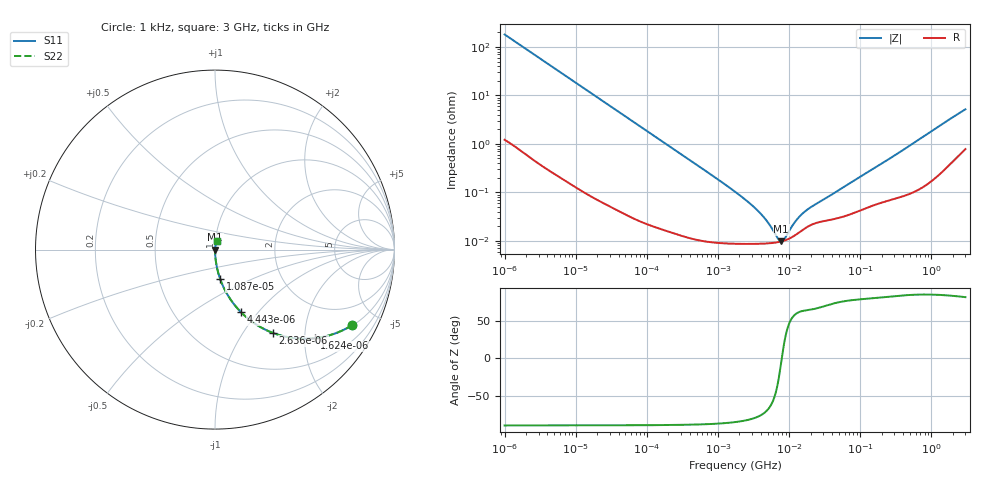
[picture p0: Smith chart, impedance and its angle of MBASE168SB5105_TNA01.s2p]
! MBASE168SB5105_TNA01  S-PARAMETER MODEL  ( Standard Model )
! Model Generated by TAIYO YUDEN Corporation (http://www.ty-top.com)
! Version 2.0
! TAIYO YUDEN Control No. 240510
! Copyright(c) 2012 TAIYO YUDEN CO.,LTD. All Rights Reserved.
! Product Description (link to TY-COMPAS)
! https://ds.yuden.co.jp/TYCOMPAS/or/detail?pn=MBASE168SB5105KTNA01&u=M
! Products Name : Multilayer Ceramic Capacitors
! Characteristics :
!  Capacitance : 1 [uF] , Rated Voltage : 16 [V] , TCC : X5R
!  Case Size : 1.6 x 0.8 / 0.063 x 0.031 [mm/inch] , Thickness : 0.8 / 0.031 [mm/inch]
!  (Conditions: Temperature = 25 [degC] , DC Bias Voltage = 0 [V])
! External Node Assignments :
!  1  o---| |---o  2
! GND o---------o GND
! Frequency Range : 1kHz  -  3GHz  [ 401 STEP ]
# MHZ S RI R 50
! Freq[MHz].  S11 Real  S11 Imag  S21 Real  S21 Imag  S12 Real  S12 Imag  S22 Real  S22 Imag
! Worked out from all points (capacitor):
!   401 points, 1 kHz to 3 GHz, reference 50 ohm
!   read as one part in series: C = 878 nF near 1.077 kHz
!   lowest |Z| = 9.73 mohm at 7.696 MHz (marker M1)
!   series resonance near 7.883 MHz, so ESL is about 460 pH
!   S11 on the Smith chart (normalised r, x): 1 kHz: 1.02, -3.62; 1.624 kHz: 1.02, -2.24; 2.636 kHz: 1.01, -1.38; 4.443 kHz: 1.01, -0.82; 10.87 kHz: 1.00, -0.34; 3 GHz: 1.02, +0.10
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0.001  0.7647 -0.4209  0.2353 0.4209  0.2353 0.4209  0.7647 -0.4209
0.001624  0.555 -0.4936  0.445 0.4936  0.445 0.4936  0.555 -0.4936
0.002636  0.3235 -0.4646  0.6765 0.4646  0.6765 0.4646  0.3235 -0.4646
0.004443  0.1456 -0.3494  0.8544 0.3494  0.8544 0.3494  0.1456 -0.3494
0.006696  0.0706 -0.2528  0.9294 0.2528  0.9294 0.2528  0.0706 -0.2528
0.010873  0.0286 -0.1632  0.9714 0.1632  0.9714 0.1632  0.0286 -0.1632
0.01216  0.0231 -0.1468  0.9769 0.1468  0.9769 0.1468  0.0231 -0.1468
0.033275  0.00351 -0.055  0.9965 0.055  0.9965 0.055  0.00351 -0.055
0.147855  0.000336 -0.0125  0.9997 0.0125  0.9997 0.0125  0.000336 -0.0125
1.732051  8.78e-05 -0.00103  0.9999 0.00103  0.9999 0.00103  8.78e-05 -0.00103
2.812335  8.64e-05 -0.000581  0.9999 0.000581  0.9999 0.000581  8.64e-05 -0.000581
3.93371  8.69e-05 -0.000359  0.9999 0.000359  0.9999 0.000359  8.69e-05 -0.000359
5.106836  8.86e-05 -0.000214  0.9999 0.000214  0.9999 0.000214  8.86e-05 -0.000214
6.881678  9.33e-05 -6.54e-05  0.9999 6.54e-05  0.9999 6.54e-05  9.33e-05 -6.54e-05
7.696136  9.66e-05 -1.14e-05  0.9999 1.14e-05  0.9999 1.14e-05  9.66e-05 -1.14e-05
8.606987  0.000101 4.24e-05  0.9999 -4.24e-05  0.9999 -4.24e-05  0.000101 4.24e-05
11.59828  0.000125 0.000188  0.9999 -0.000188  0.9999 -0.000188  0.000125 0.000188
13.97519  0.00015 0.000279  0.9998 -0.000279  0.9998 -0.000279  0.00015 0.000279
21.06097  0.000218 0.000466  0.9998 -0.000466  0.9998 -0.000466  0.000218 0.000466
256.0921  0.000705 0.00487  0.9993 -0.00487  0.9993 -0.00487  0.000705 0.00487
1780.008  0.00462 0.0314  0.9954 -0.0314  0.9954 -0.0314  0.00462 0.0314
3000  0.0103 0.0501  0.9897 -0.0501  0.9897 -0.0501  0.0103 0.0501
